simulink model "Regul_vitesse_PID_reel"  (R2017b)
settings: Solver=ode5  StartTime=0.0  StopTime=inf  FixedStep=0.005  RelTol=1e-3  AbsTol=1e-6
undefined symbols (not defined in the file or in its folder): RTDAC4PCIBaseAddress

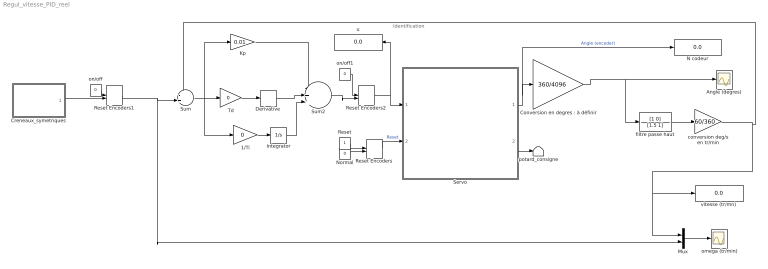
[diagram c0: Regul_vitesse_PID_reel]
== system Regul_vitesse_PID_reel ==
  note: Identification
  " omega (tr/min)" : Scope
  1/Ti : Gain  Gain=0
  Angle (degres) : Scope
  "Conversion en degres : à définir" : Gain  Gain=360/4096
  Creneaux_symetriques : Subsystem
  Derivative : Derivative
  Integrator : Integrator
  Kp : Gain  Gain=0.01
  Mux : Mux  Inputs=2
  N codeur : Display
  Normal : Constant  Value=0
  Reset : Constant
  Reset Encoders : ManualSwitch  CurrentSetting=0
  Reset Encoders1 : ManualSwitch  CurrentSetting=0
  Reset Encoders2 : ManualSwitch  CurrentSetting=0
  Servo : Subsystem  mask{BaseAddress=RTDAC4PCIBaseAddress(-1,-1), T0=0.005}
      mask prompts: BaseAddress "Base Address:"; T0 "Sampling Period:"
  Sum : Sum  Inputs=-+|
  Sum2 : Sum  Inputs=|+||+|+||
  Td : Gain  Gain=0
  conversion deg/s en tr/min : Gain  Gain=60/360
  filtre passe haut : TransferFcn  Numerator=[1 0]  Denominator=[1.5 1]
  on/off : Constant  Value=0
  on/off1 : Constant  Value=0
  potard_consigne : Terminator
  u : Display
  vitesse (tr/mn) : Display
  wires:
  Reset Encoders/1 -> Servo/2(Reset Encoder)  "Reset"
  Normal/1 -> Reset Encoders/2
  Reset/1 -> Reset Encoders/1
  Servo/2(Set-up) -> potard_consigne/1
  Servo/1(Codeur_angulaire) -> N codeur/1, "Conversion en degres : à définir"/1  "Angle (encoder)"
  Mux/1 -> " omega (tr/min)"/1
  on/off/1 -> Reset Encoders1/1
  Creneaux_symetriques/1(u) -> Reset Encoders1/2
  Reset Encoders1/1 -> Mux/2, Sum/2
  Integrator/1 -> Sum2/3
  Derivative/1 -> Sum2/2
  Kp/1 -> Sum2/1
  1/Ti/1 -> Integrator/1
  Sum/1 -> 1/Ti/1, Kp/1, Td/1
  "Conversion en degres : à définir"/1 -> filtre passe haut/1, Angle (degres)/1
  Sum2/1 -> Reset Encoders2/2
  on/off1/1 -> Reset Encoders2/1
  conversion deg/s en tr/min/1 -> Mux/1, vitesse (tr/mn)/1, Sum/1
  Reset Encoders2/1 -> u/1, Servo/1(PWM Control)
  filtre passe haut/1 -> conversion deg/s en tr/min/1
  Td/1 -> Derivative/1

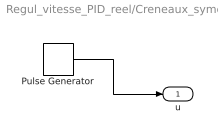
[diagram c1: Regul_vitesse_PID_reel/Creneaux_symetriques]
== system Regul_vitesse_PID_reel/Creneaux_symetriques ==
  Pulse Generator : DiscretePulseGenerator  PulseType=Time based  Amplitude=500  Period=0.005*floor(15/0.005)  PulseWidth=50  PhaseDelay=0.005*floor(0*15/0.005/4)
  u : Outport
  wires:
  Pulse Generator/1 -> u/1

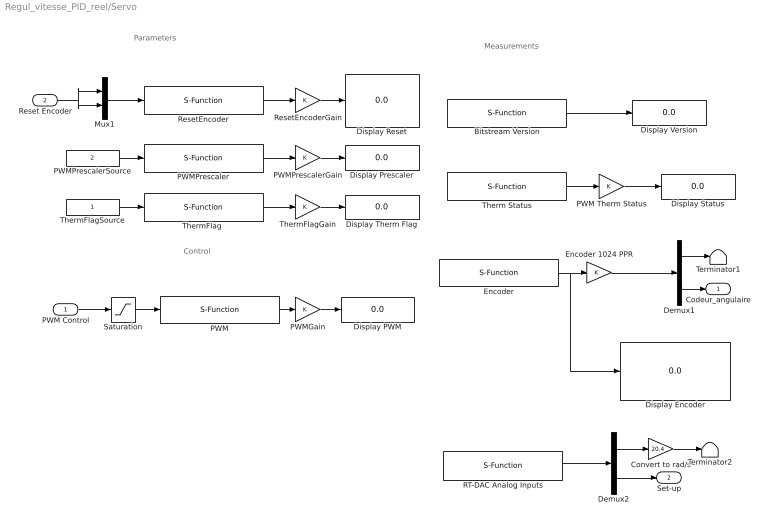
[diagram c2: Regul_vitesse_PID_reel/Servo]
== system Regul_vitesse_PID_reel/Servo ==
  note: Parameters
  note: Control
  note: Measurements
  PWM Control : Inport
  Reset Encoder : Inport  Port=2
  Bitstream Version : S-Function  FunctionName=Servo_BitstreamVersion  Parameters=BaseAddress, T0  SFunctionDeploymentMode=off  EnableBusSupport=off
  Convert to rad/s : Gain  Gain=20.4
  Demux1 : Demux  Outputs=2
  Demux2 : Demux  Outputs=2
  Display Encoder : Display
  Display PWM : Display
  Display Prescaler : Display
  Display Reset : Display
  Display Status : Display
  Display Therm Flag : Display
  Display Version : Display
  Encoder : S-Function  FunctionName=Servo_Encoder  Parameters=BaseAddress, T0  SFunctionDeploymentMode=off  EnableBusSupport=off
  Encoder 1024 PPR : Gain
  Mux1 : Mux  Inputs=2
  PWM : S-Function  FunctionName=Servo_PWM  Parameters=BaseAddress, T0  SFunctionDeploymentMode=off  EnableBusSupport=off
  PWM Therm Status : Gain
  PWMGain : Gain
  PWMPrescaler : S-Function  FunctionName=Servo_PWMPrescaler  Parameters=BaseAddress, T0  SFunctionDeploymentMode=off  EnableBusSupport=off
  PWMPrescalerGain : Gain
  PWMPrescalerSource : Constant  Value=2
  RT-DAC Analog Inputs : S-Function  FunctionName=servo_analoginputs  Parameters=BaseAddress, [1 0], [1 1], T0  SFunctionDeploymentMode=off  EnableBusSupport=off
  ResetEncoder : S-Function  FunctionName=Servo_ResetEncoder  Parameters=BaseAddress, T0  SFunctionDeploymentMode=off  EnableBusSupport=off
  ResetEncoderGain : Gain
  Saturation : Saturate  UpperLimit=1  LowerLimit=-1
  Terminator1 : Terminator
  Terminator2 : Terminator
  Therm Status : S-Function  FunctionName=Servo_PWMTherm  Parameters=BaseAddress, T0  SFunctionDeploymentMode=off  EnableBusSupport=off
  "ThermFlag " : S-Function  FunctionName=Servo_ThermFlag  Parameters=BaseAddress, T0  SFunctionDeploymentMode=off  EnableBusSupport=off
  ThermFlagGain : Gain
  ThermFlagSource : Constant
  Codeur_angulaire : Outport
  Set-up : Outport  Port=2
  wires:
  Encoder/1 -> Encoder 1024 PPR/1, Display Encoder/1
  Saturation/1 -> PWM/1
  PWM/1 -> PWMGain/1
  PWMGain/1 -> Display PWM/1
  ResetEncoder/1 -> ResetEncoderGain/1
  PWMPrescaler/1 -> PWMPrescalerGain/1
  Mux1/1 -> ResetEncoder/1
  PWMPrescalerSource/1 -> PWMPrescaler/1
  ResetEncoderGain/1 -> Display Reset/1
  PWMPrescalerGain/1 -> Display Prescaler/1
  PWM Control/1 -> Saturation/1
  Encoder 1024 PPR/1 -> Demux1/1
  Therm Status/1 -> PWM Therm Status/1
  PWM Therm Status/1 -> Display Status/1
  Bitstream Version/1 -> Display Version/1
  Reset Encoder/1 -> Mux1/1, Mux1/2
  "ThermFlag "/1 -> ThermFlagGain/1
  ThermFlagSource/1 -> "ThermFlag "/1
  ThermFlagGain/1 -> Display Therm Flag/1
  Demux1/1 -> Terminator1/1
  Demux1/2 -> Codeur_angulaire/1
  RT-DAC Analog Inputs/1 -> Demux2/1
  Demux2/2 -> Set-up/1
  Demux2/1 -> Convert to rad/s/1
  Convert to rad/s/1 -> Terminator2/1
